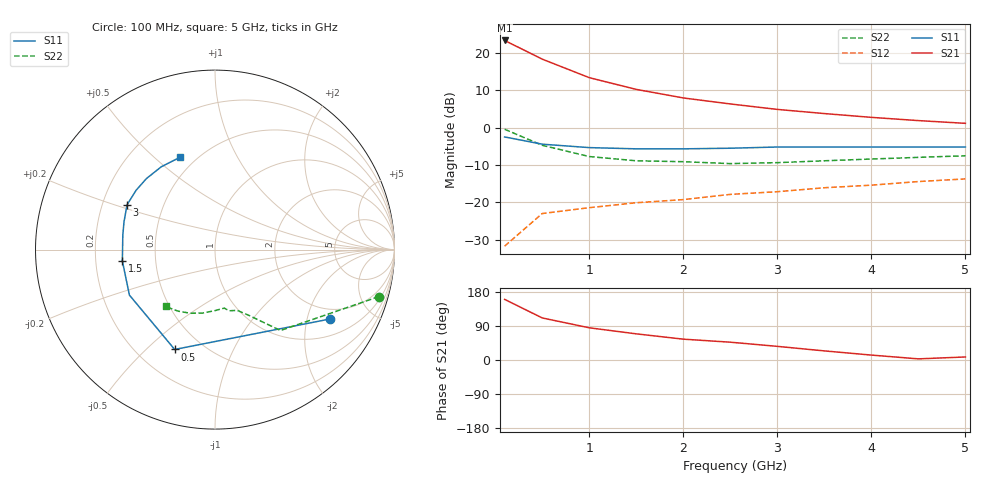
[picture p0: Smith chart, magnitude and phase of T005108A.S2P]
!AT-00510
!S-PARAMETERS at Vce=8V  Ic=5mA.  LAST UPDATED 07-21-92
!OBSOLETED Feb 1994 - nearest replacement: AT-41410
# ghz s ma r 50
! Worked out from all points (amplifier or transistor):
!   11 points, 100 MHz to 5 GHz, reference 50 ohm
!   highest |S21| = 23.3 dB at 100 MHz (marker M1)
!   |S21| within 3 dB of that: start of sweep to 340.2 MHz
!   unconditionally stable (mu >= 1): 1.599 GHz to end of sweep
!   at 500 MHz: K = 0.41, MSG = 20.6 dB, |S12| = -23.0 dB
!   at 2.5 GHz: K = 1.17, MAG = 9.6 dB, |S12| = -17.9 dB
!   at 5 GHz: K = 1.19, MAG = 4.8 dB, |S12| = -13.7 dB
!   S11 on the Smith chart (normalised r, x): 100 MHz: 1.58, -2.79; 500 MHz: 0.35, -0.61; 1.5 GHz: 0.32, -0.06; 3 GHz: 0.31, +0.22; 5 GHz: 0.41, +0.61
0.1  0.75 -31.0  14.61 160.0  0.026 81.0  0.95 -16.0
0.5  0.6 -112.0  8.22 111.0  0.071 42.0  0.58 -51.0
1  0.54 -152.0  4.65 85.0  0.085 33.0  0.41 -63.0
1.5  0.52 -173.0  3.24 69.0  0.099 33.0  0.36 -70.0
2  0.52 171.0  2.49 55.0  0.109 33.0  0.35 -77.0
2.5  0.53 163.0  2.07 47.0  0.128 35.0  0.33 -81.0
3  0.55 153.0  1.75 36.0  0.139 36.0  0.34 -90.0
3.5  0.55 143.0  1.54 24.0  0.157 32.0  0.36 -101.0
4  0.55 134.0  1.37 13.0  0.17 30.0  0.38 -111.0
4.5  0.55 123.0  1.24 3.0  0.19 25.0  0.4 -121.0
5  0.55 111.0  1.14 8.0  0.206 20.0  0.42 -131.0
